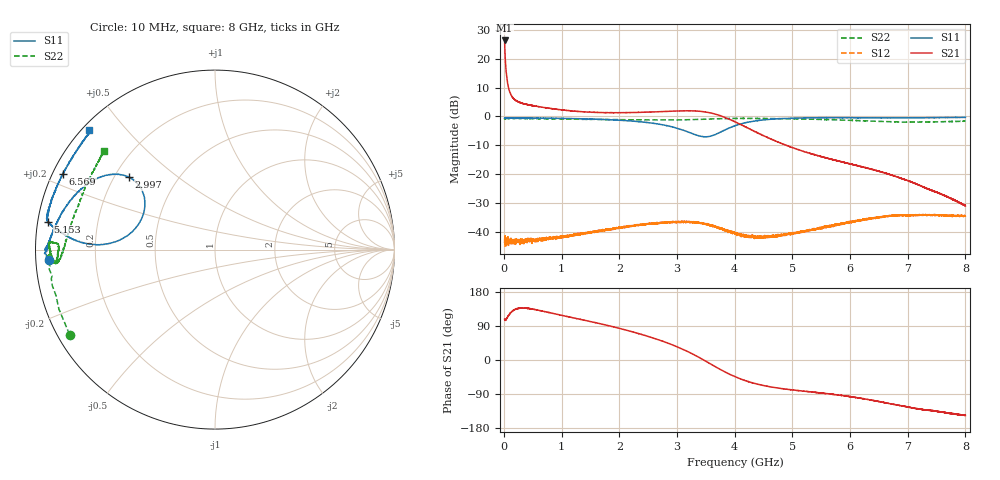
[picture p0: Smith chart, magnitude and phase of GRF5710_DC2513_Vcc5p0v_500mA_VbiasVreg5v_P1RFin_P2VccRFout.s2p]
!Keysight Technologies,N5244B,MY57181157,A.18.40.03
!Date: Thursday, September 18, 2025 15:49:23
!Correction: S11(C  2-Port  )
!S21(C  2-Port  )
!S12(C  2-Port  )
!S22(C  2-Port  )
!S2P File: Measurements: S11, S21, S12, S22:
# Hz S  RI  R 50
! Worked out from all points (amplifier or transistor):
!   7991 points, 10 MHz to 8 GHz, reference 50 ohm
!   highest |S21| = 26.4 dB at 10 MHz (marker M1)
!   |S21| within 3 dB of that: start of sweep to 14.21 MHz
!   unconditionally stable (mu >= 1): 124.6 MHz to 127.6 MHz; 128.2 MHz to 144 MHz; 144 MHz to end of sweep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
!   at 1.341 GHz: K = 1.94, MAG = 15.6 dB, |S12| = -40.6 dB
!   at 4.005 GHz: K = 5.80, MAG = 8.8 dB, |S12| = -40.7 dB
!   at 8 GHz: K = 19.34, MAG = -14.0 dB, |S12| = -34.8 dB
!   S11 on the Smith chart (normalised r, x): 10 MHz: 0.04, -0.03; 2.997 GHz: 0.26, +0.34; 5.153 GHz: 0.03, +0.08; 6.569 GHz: 0.03, +0.24; 8 GHz: 0.02, +0.40
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1e7  -0.9268 -0.059  -6.542 19.86  0.00636 5.85e-05  -0.81 -0.4739
5e7  -0.9376 -0.0102  -1.561 4.265  0.00772 -7.15e-05  -0.9269 -0.0974
5.5e7  -0.9375 -4.59e-06  -1.504 3.858  0.00713 0.00156  -0.9198 -0.0924
6.1e7  -0.9428 -0.0131  -1.549 3.527  0.00649 -0.000242  -0.9258 -0.0865
7.3e7  -0.9416 -0.00258  -1.456 2.998  0.00662 1.18e-05  -0.9261 -0.0687
9e7  -0.9408 0.00144  -1.427 2.483  0.00701 -0.000283  -0.9292 -0.0635
1.13e8  -0.9395 0.00289  -1.372 2.033  0.0059 0.000329  -0.923 -0.0484
1.42e8  -0.9396 0.00149  -1.372 1.722  0.00699 0.000795  -0.9307 -0.0397
2.21e8  -0.9421 0.00693  -1.304 1.312  0.00688 0.000651  -0.9228 -0.0303
3.52e8  -0.9398 0.00681  -1.216 1.131  0.00702 0.00134  -0.9263 -0.0358
1.342e9  -0.908 0.0867  -0.3458 1.161  0.00888 0.00219  -0.8903 -0.0716
2.674e9  -0.6136 0.4118  0.7179 0.9718  0.0131 -0.00394  -0.8714 0.00519
2.997e9  -0.4797 0.4046  1.017 0.7154  0.012 -0.00841  -0.8729 0.0266
3.478e9  -0.4033 0.1856  1.201 -0.0298  0.00147 -0.0136  -0.8949 0.0391
3.751e9  -0.5314 0.0533  0.9337 -0.4359  -0.00577 -0.01  -0.9132 0.0414
4.005e9  -0.6915 0.0298  0.5804 -0.5619  -0.00847 -0.00375  -0.9217 0.04
4.458e9  -0.8568 0.0948  0.1978 -0.4417  -0.00747 0.00331  -0.92 0.0105
5.153e9  -0.9302 0.1552  0.0373 -0.2527  -0.00388 0.00891  -0.9006 -0.0595
5.337e9  -0.9369 0.1649  0.0217 -0.2229  -0.00363 0.0101  -0.8932 -0.0705
6.569e9  -0.8462 0.4235  -0.0393 -0.0996  0.00403 0.0175  -0.8118 0.1124
6.669e9  -0.8289 0.4544  -0.0415 -0.0906  0.00517 0.0182  -0.8014 0.1487
8e9  -0.6999 0.6674  -0.0234 -0.0154  0.0118 0.0137  -0.6197 0.5489
